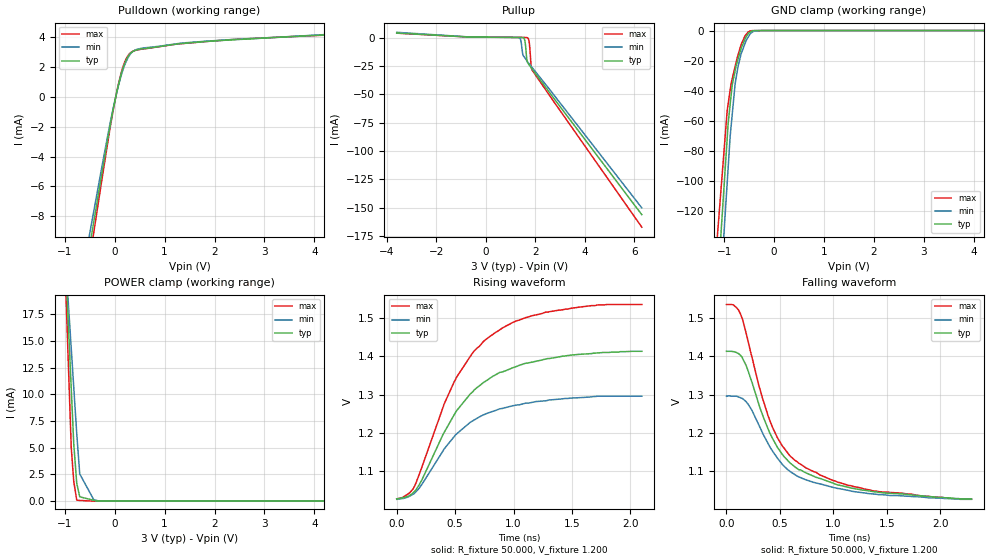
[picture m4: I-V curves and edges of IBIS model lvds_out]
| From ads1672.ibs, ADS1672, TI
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[Model]   lvds_out
Model_type Output
Vref=1.200E+00
Rref=5.000E+02
Cref=5.000E-12
Vmeas=1.200E+00
C_comp   1.220E-12   1.220E-12   1.220E-12
[Voltage Range]   3.000E+00   2.700E+00   3.300E+00
[POWER Clamp Reference]   3.000E+00   2.700E+00   3.300E+00
[GND Clamp Reference]   0.000E+00   0.000E+00   0.000E+00
[Pullup Reference]   3.000E+00   2.700E+00   3.300E+00
[Pulldown Reference]   0.000E+00   0.000E+00   0.000E+00
[Temperature Range]   25   85   -40
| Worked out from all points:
|   slope of the pulldown table from 0 to 0.45 V, typ, clamps not added: 128 ohm
|   slope of the pullup table from 0 to 0.45 V, typ, clamps not added: 5.81 kohm
|   GND clamp passes 1 mA (typ) near -0.48 V on its own axis
|   POWER clamp passes 1 mA (typ) near -0.73 V on its own axis
|   rising waveform, R_fixture 50.000, V_fixture 1.200: 20-80 % time 508ps typ, 463ps min, 492ps max; typ from 1.03 V to 1.41 V
|   falling waveform, R_fixture 50.000, V_fixture 1.200: 20-80 % time 439ps typ, 449ps min, 430ps max; typ from 1.41 V to 1.03 V
[GND Clamp]
-3.3V     -1.275A    -1.329A    -1.054A
-2.7V     -968.8mA   -1.017A    -799.8mA
-940mV    -71.79mA   -101.4mA   -53.33mA
-920mV    -61.6mA    -91mA      -48.74mA
-880mV    -49.03mA   -70.19mA   -39.56mA
-840mV    -36.47mA   -56.19mA   -32.19mA
-780mV    -26.62mA   -35.18mA   -23.81mA
-660mV    -11.74mA   -15.44mA   -9.272mA
-580mV    -5.555mA   -8.396mA   -3.409mA
-480mV    -1.027mA   -2.221mA   -318uA
-190mV    0A         0A         0A
6.6V      0A         0A         0A
[Power Clamp]
-3.6V     293.6mA    212mA      405.6mA
-1.06V    30.26mA    28.05mA    30.66mA
-870mV    10.56mA    14.3mA     5.022mA
-820mV    5.376mA    10.68mA    1.862mA
-760mV    1.674mA    6.334mA    94.53uA
-700mV    403.2uA    2.546mA    64.68uA
-420mV    80.64uA    139.4uA    0A
-320mV    0A         12.67uA    0A
6.3V      0A         0A         0A
[Pullup]
-3.6V     4.01mA     4.6mA      3.87mA
-740mV    534uA      613uA      521uA
1.36V     102uA      -278uA     133uA
1.42V     88.1uA     -3.33mA    122uA
1.5V      -52.6uA    -15.4mA    107uA
1.58V     -3.21mA    -18mA      90.5uA
1.66V     -20.1mA    -20.5mA    -21uA
1.7V      -22.6mA    -21.8mA    -490uA
1.76V     -24.4mA    -23.4mA    -5.46mA
1.82V     -26.2mA    -25mA      -22.8mA
1.86V     -27.4mA    -26.1mA    -28.3mA
6.3V      -156mA     -150mA     -167mA
[Pulldown]
-3.3V     -65.92mA   -60.35mA   -71.53mA
-320mV    -6.392mA   -5.852mA   -6.936mA
-60mV     -1.359mA   -1.244mA   -1.463mA
20mV      -23.1uA    -11.5uA    -18.9uA
100mV     1.13mA     1.07mA     1.21mA
160mV     1.85mA     1.75mA     1.95mA
240mV     2.53mA     2.44mA     2.62mA
320mV     2.93mA     2.9mA      2.97mA
400mV     3.11mA     3.12mA     3.11mA
1.38V     3.59mA     3.62mA     3.58mA
2.38V     3.83mA     3.85mA     3.85mA
6.6V      4.58mA     4.62mA     4.48mA
[Rising Waveform]
R_fixture = 50.000
V_fixture = 1.200
V_fixture_min = 1.200
V_fixture_max = 1.200
|  time   V(typ)   V(min)   V(max)
0s        1.028V     1.027V     1.028V
152.5ps   1.047V     1.043V     1.061V
405ps     1.201V     1.158V     1.275V
492.5ps   1.248V     1.191V     1.334V
662.5ps   1.312V     1.234V     1.414V
780ps     1.339V     1.252V     1.448V
992ps     1.37V      1.271V     1.488V
1.275ns   1.393V     1.284V     1.515V
1.722ns   1.409V     1.296V     1.534V
2.097ns   1.413V     1.296V     1.535V
[Falling Waveform]
R_fixture = 50.000
V_fixture = 1.200
V_fixture_min = 1.200
V_fixture_max = 1.200
|  time   V(typ)   V(min)   V(max)
0s        1.413V     1.296V     1.535V
65ps      1.412V     1.296V     1.534V
130ps     1.403V     1.292V     1.511V
225ps     1.343V     1.265V     1.412V
390ps     1.21V      1.172V     1.244V
525ps     1.143V     1.117V     1.165V
642.5ps   1.111V     1.091V     1.128V
997.5ps   1.069V     1.058V     1.076V
1.285ns   1.051V     1.044V     1.054V
2.29ns    1.028V     1.027V     1.028V
[Ramp]
dV/dt_f   2.4209E+00/4.4527E-10   2.2438E+00/4.4826E-10   2.5997E+00/4.2922E-10
dV/dt_r   2.4209E+00/5.0320E-10   2.2438E+00/4.6770E-10   2.5997E+00/4.9030E-10
R_load = 50
